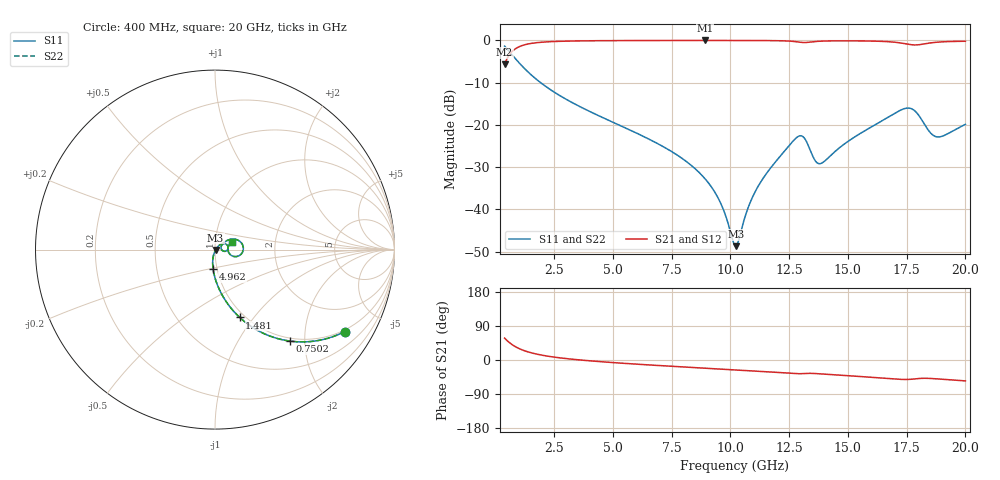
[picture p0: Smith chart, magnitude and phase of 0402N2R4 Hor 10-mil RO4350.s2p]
# GHz S MA R 50
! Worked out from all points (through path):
!   1960 points, 400 MHz to 20 GHz, reference 50 ohm
!   highest |S21| = -0.03 dB at 8.924 GHz (marker M1); lowest = -5.7 dB at 400 MHz (marker M2)
!   group delay of S21, straight-line fit = 11.1 ps
!   lowest |S11| = -48.7 dB at 10.24 GHz (marker M3), VSWR 1.01, Z = 50.3 - j0.17 ohm
!   |S11| at or under -10 dB: 1.93 GHz to end of sweep
!   |S22| runs from -48.7 to -1.4 dB; largest |S21 - S12| = 0
!   S11 on the Smith chart (normalised r, x): 400 MHz: 0.94, -3.20; 750.2 MHz: 0.94, -1.70; 1.481 GHz: 0.95, -0.85; 4.962 GHz: 0.96, -0.21; 20 GHz: 1.20, +0.10
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0.4  0.8549 -32.3  0.5185 57.7  0.5185 57.7  0.8549 -32.3
0.7501787  0.659 -50.7  0.7515 39.3  0.7515 39.3  0.659 -50.7
1.070342  0.5218 -61.2  0.8522 28.7  0.8522 28.7  0.5218 -61.2
1.480551  0.402 -70.0  0.9146 19.9  0.9146 19.9  0.402 -70.0
3.671669  0.1608 -89.7  0.9851 -0.3  0.9851 -0.3  0.1608 -89.7
4.962328  0.1089 -95.5  0.9918 -6.6  0.9918 -6.6  0.1089 -95.5
6.943338  0.05941 -102.2  0.9955 -14.5  0.9955 -14.5  0.05941 -102.2
8.924349  0.0231 -104.2  0.9963 -21.6  0.9963 -21.6  0.0231 -104.2
9.594691  0.0118 -97.8  0.9962 -24.0  0.9962 -24.0  0.0118 -97.8
10.205  0.00371 -35.6  0.9959 -26.1  0.9959 -26.1  0.00371 -35.6
10.23502  0.003683 -27.3  0.9959 -26.2  0.9959 -26.2  0.003683 -27.3
11.00541  0.01518 43.5  0.9949 -29.0  0.9949 -29.0  0.01518 43.5
12.06595  0.04088 43.6  0.9892 -33.0  0.9892 -33.0  0.04088 43.6
12.96641  0.07434 13.4  0.9497 -36.2  0.9497 -36.2  0.07434 13.4
13.18652  0.06755 -3.4  0.9416 -35.6  0.9416 -35.6  0.06755 -3.4
13.46667  0.04525 -9.8  0.9584 -35.3  0.9584 -35.3  0.04525 -9.8
13.67677  0.03595 1.9  0.9708 -35.9  0.9708 -35.9  0.03595 1.9
13.89689  0.03542 17.6  0.9784 -36.9  0.9784 -36.9  0.03542 17.6
16.73834  0.1247 27.6  0.9628 -48.9  0.9628 -48.9  0.1247 27.6
17.70883  0.1553 -3.8  0.8868 -50.7  0.8868 -50.7  0.1553 -3.8
18.80939  0.07207 -0.5  0.9508 -49.9  0.9508 -49.9  0.07207 -0.5
20  0.1015 24.0  0.9752 -55.1  0.9752 -55.1  0.1015 24.0
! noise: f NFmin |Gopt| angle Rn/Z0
0.4  0.00126  0.793  3.697  0.001255
2.571  0.005073  0.6794  7.751  0.003045
4.752  0.008086  0.6384  13.01  0.004167
6.933  0.01087  0.6157  18.32  0.005134
9.104  0.01384  0.6092  23.55  0.006304
11.29  0.01972  0.6547  28.73  0.01024
13.47  0.06005  0.8509  34.15  0.07844
15.64  0.03553  0.7308  39.13  0.02342
17.82  0.1172  0.8998  44.42  0.2193
20  0.04858  0.7542  49.18  0.03314
